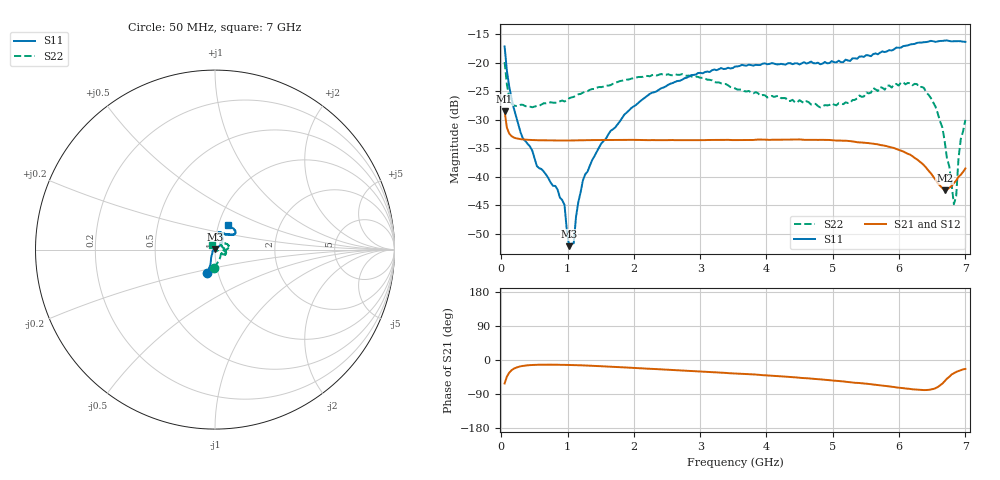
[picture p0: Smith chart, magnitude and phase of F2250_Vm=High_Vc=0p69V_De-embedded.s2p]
! Integrated Device Technology
! Corporate Headquarters
! 6024 Silver Creek Valley Road
! San Jose, CA 95138  USA
! Phone:  1-408-284-8200
! Toll Free:  1-800-223-1366
! Webpage:  http://www.idt.com/
! Timing and RF Division
! 515 Groton Road, Suite 102
! Westford, MA 01886-6024
! Device:  F2250
! Description: Voltage Variable RF Attenuator
! Frequency:  50.0 -  6000.00 MHz
! Package:  3x3 mm Thin QFN Plastic Package: 16 pin
! Ports:  2 RF, 3 DC
!  Pin  1  = GND
!  Pin  2  = NC
!  Pin  3  = RF1  = Port 1
!  Pin  4  = NC
!  Pin  5  = GND
!  Pin  6  = GND
!  Pin  7  = GND
!  Pin  8  = GND
!  Pin  9  = NC
!  Pin 10  = RF2  = Port 2
!  Pin 11  = NC
!  Pin 12  = GND
!  Pin 13  = GND
!  Pin 14  = VCNTRL
!  Pin 15  = VDD
!  Pin 16  = VMODE
! Vcntrl:  0.690 Volts
! Vmode:  +3.300 Volts
! Vdd:  +3.30  Volts
! Current:  1.286 mA
! Data:  The device was measured on a the F2250 evaluation board which has
!  individual transmission lines to the RF pins.  Data was collected
!  using a calibrated network analyzer.  The evaluation board was
!  de-embedded using a TRL calibration technique.
!  The reference plane is the edge of the package pin.
! Misc:  SN 10
!  Action Tracker AT0258
! Date Measured:  2014-11-26
! Date:  2015-10-15  MJV
! Note:
!  Integrated Device Technology supplies this data as a sample of measured
!  data at the package pin for this product.  Your particular data for this
!  product may vary.
!  Data was taken at 25 degrees C.
!  Integrated Device Technology reserves the right to change this data at anytime.
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# GHz S dB R 50
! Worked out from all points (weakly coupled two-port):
!   201 points, 50 MHz to 7 GHz, reference 50 ohm
!   highest |S21| = -28.51 dB at 50 MHz (marker M1); lowest = -42.4 dB at 6.687 GHz (marker M2)
!   lowest |S11| = -52.2 dB at 1.023 GHz (marker M3), VSWR 1.00, Z = 49.8 + j0.169 ohm
!   |S11| at or under -10 dB: start of sweep to end of sweep
!   |S22| runs from -44.8 to -19.9 dB; largest |S21 - S12| = 6.2e-05
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0.05  -17.16 -108.2  -28.51 -61.8  -28.50 -61.8  -19.90 -93.1
0.1195  -24.20 -111.4  -32.45 -33.4  -32.44 -33.3  -26.10 -52.9
0.189  -28.02 -119.2  -33.14 -23.0  -33.14 -23.0  -27.53 -35.4
0.5365  -38.14 -153.1  -33.61 -12.7  -33.62 -12.6  -27.60 -8.8
0.9535  -44.96 171.7  -33.68 -12.8  -33.68 -12.9  -26.82 -5.1
1.023  -52.20 136.2  -33.66 -13.1  -33.66 -13.1  -26.27 -4.1
1.0925  -51.70 78.2  -33.65 -13.4  -33.65 -13.4  -26.01 -3.3
1.12725  -47.03 55.0  -33.65 -13.6  -33.64 -13.6  -25.76 -3.8
1.2315  -40.62 37.7  -33.62 -14.2  -33.62 -14.2  -25.26 -4.4
1.6485  -31.97 40.1  -33.58 -17.6  -33.59 -17.6  -23.95 1.4
2.37825  -24.74 46.2  -33.59 -24.4  -33.58 -24.4  -22.13 10.4
3.525  -20.68 71.5  -33.59 -35.5  -33.59 -35.5  -24.51 35.3
4.7065  -20.10 71.8  -33.53 -49.6  -33.54 -49.6  -27.23 42.3
5.85325  -17.81 40.4  -34.79 -69.7  -34.79 -69.8  -24.02 -10.5
6.3745  -16.42 40.8  -37.99 -79.3  -37.99 -79.4  -24.42 -26.9
6.54825  -16.36 44.5  -40.53 -74.5  -40.54 -74.5  -27.69 -33.6
6.68725  -16.13 47.7  -42.41 -56.0  -42.42 -55.9  -33.77 -22.9
6.82625  -16.25 52.4  -41.14 -34.9  -41.11 -34.9  -44.84 72.3
6.861  -16.24 54.3  -40.69 -31.6  -40.67 -31.7  -43.44 91.4
6.89575  -16.23 56.3  -40.04 -29.1  -40.02 -29.0  -36.87 99.5
6.9305  -16.25 58.6  -39.68 -27.0  -39.64 -27.0  -33.40 119.3
7  -16.35 62.3  -38.56 -23.4  -38.54 -23.5  -30.04 122.8
